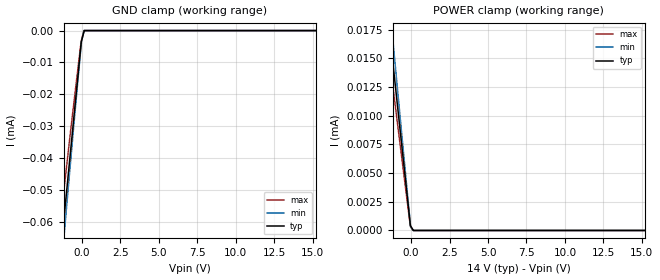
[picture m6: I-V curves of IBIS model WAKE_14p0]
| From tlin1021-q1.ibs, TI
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|   WAKE_14p0
[Model]   WAKE_14p0
Model_type   Input
Vinl = 11
Vinh = 12
|   typ   min   max
C_comp   3.243pF   3.243pF   3.4pF
[Voltage Range]   14   12   16
[Temperature Range]   25   165   -55
[Power Clamp Reference]   14   12   16
[GND Clamp Reference]   0   0   0
[GND Clamp]
|   Voltage   I(typ)   I(min)   I(max)
-14V      -714.2uA   -809.8uA   -625.3uA
-1.771V   -88.58uA   -98.13uA   -75.96uA
-1.434V   -71.95uA   -79.33uA   -61.36uA
-1.22V    -61.43uA   -67.51uA   -52.11uA
-1.095V   -55.23uA   -60.55uA   -46.7uA
-500.3mV  -25.91uA   -28.06uA   -21.57uA
-46.38mV  -3.532uA   -4.235uA   -3.172uA
-29.91mV  -3.234uA   -3.384uA   -2.879uA
130mV     -335.7nA   0A         -32.51nA
148.6mV   0A         0A         0A
28V       0A         0A         0A
[POWER Clamp]
|   Voltage   I(typ)   I(min)   I(max)
-14V      176.2uA    201.4uA    153.8uA
-1.771V   21.89uA    24.9uA     18.98uA
-1.35V    16.66uA    18.91uA    14.39uA
-1.263V   15.57uA    17.67uA    13.44uA
-1.178V   14.51uA    16.45uA    12.5uA
-373.8mV  4.497uA    5.084uA    3.814uA
-46.38mV  420.3nA    518.9nA    378.6nA
-29.91mV  384.8nA    290.2nA    343.6nA
130mV     39.94nA    0A         3.88nA
28V       0A         0A         0A
